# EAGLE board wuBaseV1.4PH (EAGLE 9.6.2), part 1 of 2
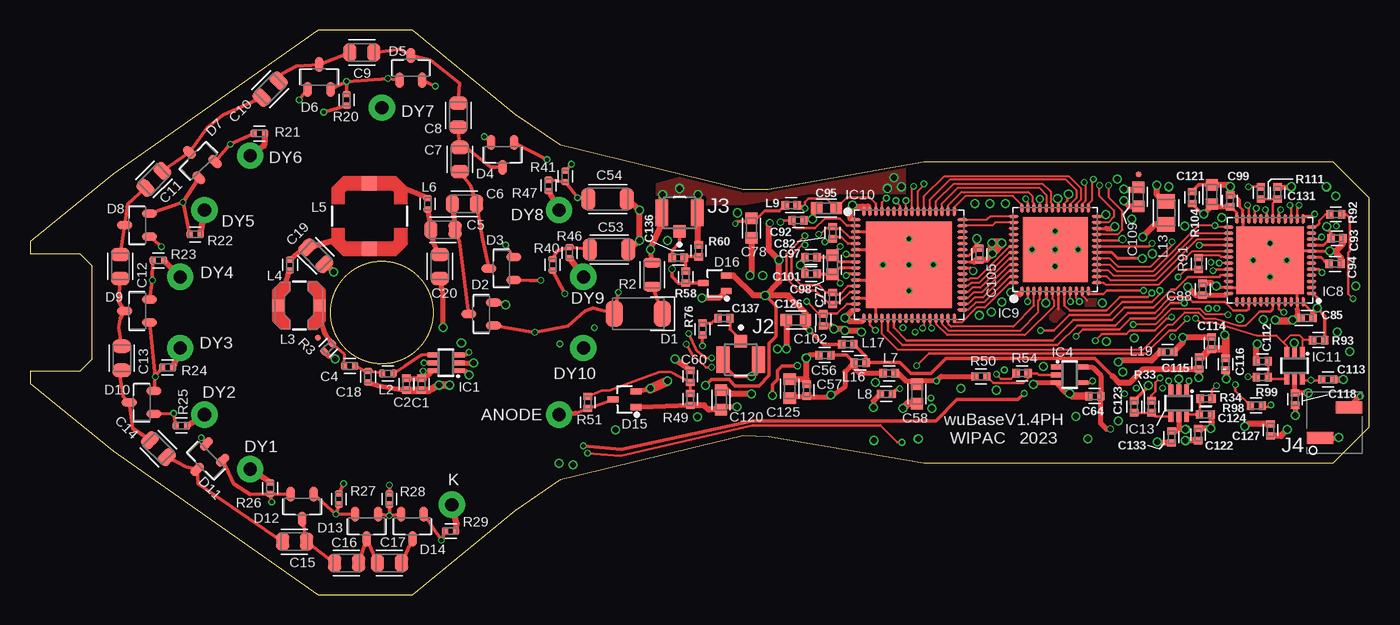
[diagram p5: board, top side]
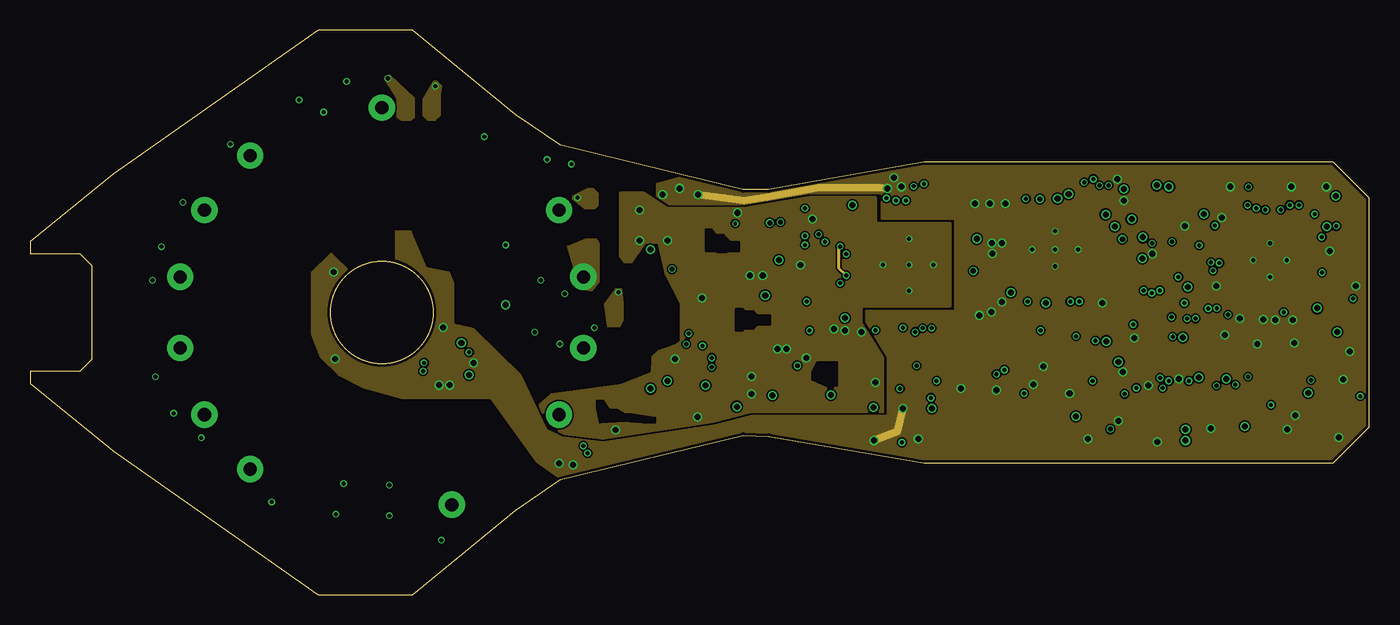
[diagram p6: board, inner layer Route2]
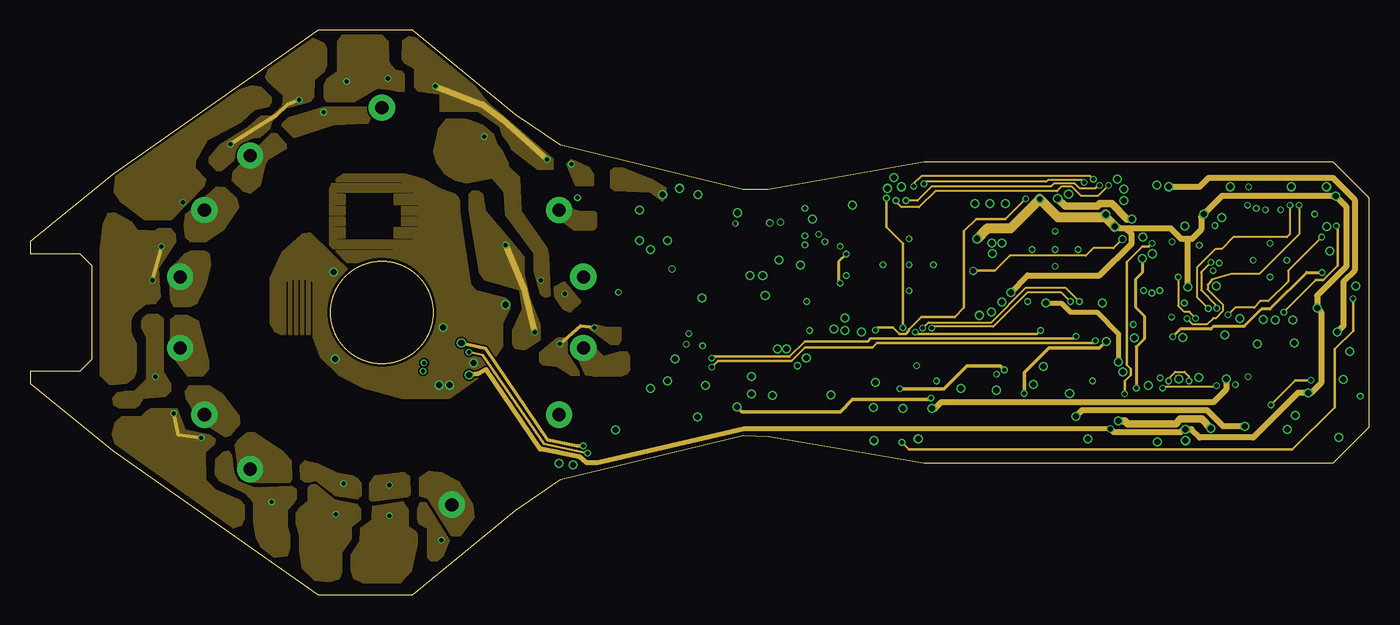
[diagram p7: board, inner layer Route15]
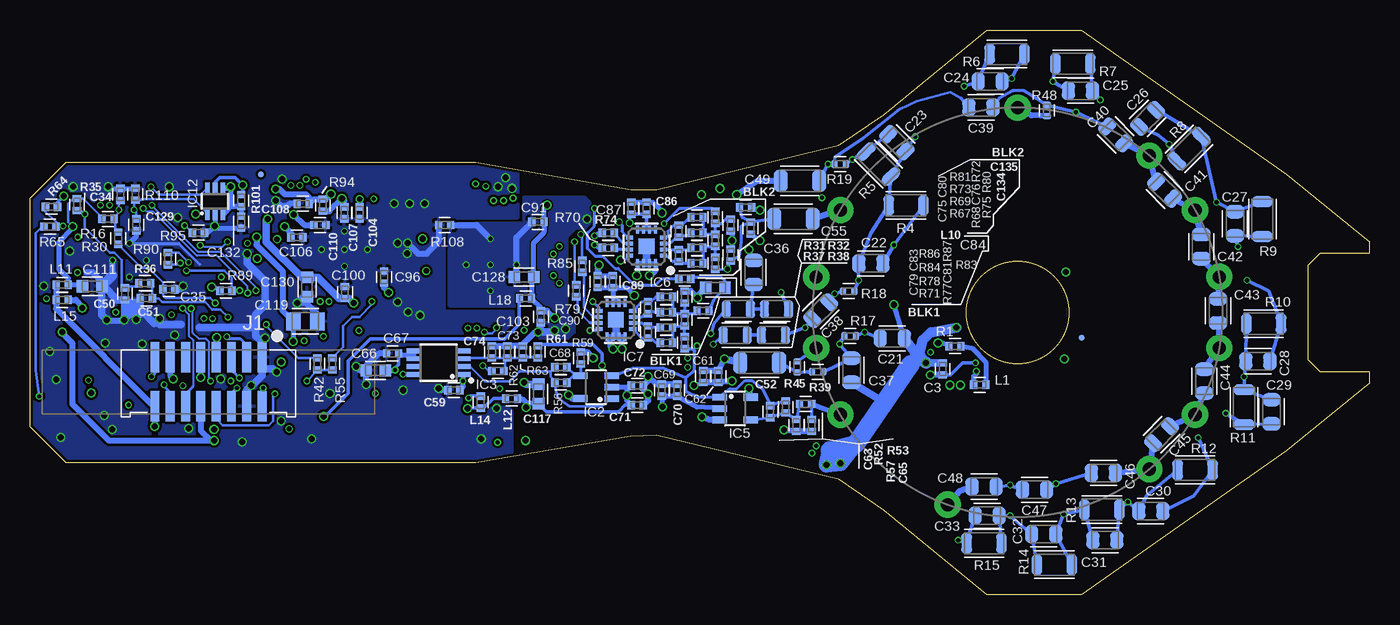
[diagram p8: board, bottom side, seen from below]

Size 111.2 x 46.9 mm. Coordinates in mm from the lower left corner, seen from the top.
Outline: 0,18.55 0,17.55 6.9,11.95 23.9,0 31.75,0 40.31,7.02 44.06,9.57 59.2,13.25 61.33,13.16 74.2,10.95 108.2,10.95 111.2,13.95 111.2,32.95 108.2,35.95 74.2,35.95 61.33,33.65 59.2,33.65 44.06,37.33 40.31,39.88 31.75,46.9 23.9,46.9 6.9,34.95 0,29.35 0,28.35 4.1,28.35 5.1,27.35 5.1,19.55 4.1,18.55 0,18.55
Outline: circle at 29.2,23.45 radius 4.25
Copper layers (1*2*15*16): Top 0.035mm / dielectric 0.23mm / Route2 0.035mm / dielectric 0.93mm / Route15 0.035mm / dielectric 0.23mm / Bottom 0.035mm
Design rules "MF_Standard_4_Layer": minimum track width 5mil, minimum drill 10mil, track to track 5mil, track to pad 5mil, pad to pad 5mil, via to via 5mil, smd to smd 0mil, copper to edge 10mil, drill to drill 10mil, minimum pad ring 4mil, minimum via ring 4mil, stop-mask expansion 2mil, vias tented up to drill 25mil, thermal gap 10mil

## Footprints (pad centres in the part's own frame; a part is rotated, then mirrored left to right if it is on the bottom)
0430-BARE = drill 1.092 pad 2.184: P$1 0,0
C0402 = smd 0.6 x 0.7: 1 -0.5,0; 2 0.5,0
C0402-HV = smd 0.56 x 0.7: 1 -0.47,0; 2 0.47,0
C0805-HV = smd 1.1 x 1.5: 1 -1,0; 2 1,0
C1206-HV = smd 1.165 x 1.815: 1 -1.6,0; 2 1.6,0
C0603 = smd 0.95 x 1: 1 -0.8,0; 2 0.8,0
C0805 = smd 1.2 x 1.5: 1 -1,0; 2 1,0
DO214AC-HV = smd 1.4 x 2.2: A 2,0; C -2,0
SOT23-ROUNDED = smd 1.242 x 0.694: 1 -1.029,0.95; 2 -1.029,-0.95; 3 1.029,0
SC70-3L = smd 0.5 x 0.9: 1 -0.65,-0.95; 2 0.65,-0.95; 3 0,0.95
FIDUCIAL_0.5MM = smd 0.5 x 0.5 bottom: FID_BOT 0,0 | smd 0.5 x 0.5: FID_TOP 0,0
SC70-6L-TI = smd 0.4 x 0.9: 1 -0.65,-1.1; 2 0,-1.1; 3 0.65,-1.1; 4 0.65,1.1; 5 0,1.1; 6 -0.65,1.1
SOT23-5 = smd 0.55 x 1.2: 1 -0.95,-1.3; 2 0,-1.3; 3 0.95,-1.3; 4 0.95,1.3 | smd 0.6 x 1.2: 5 -0.95,1.3
MSOP8 = smd 0.4 x 1.2: 1 -0.975,-2.05; 2 -0.325,-2.05; 3 0.325,-2.05; 4 0.975,-2.05; 5 0.975,2.05; 6 0.325,2.05; 7 -0.325,2.05; 8 -0.975,2.05
SC70-5L-TI = smd 0.4 x 0.9: 1 -0.65,-1.1; 2 0,-1.1; 3 0.65,-1.1; 4 0.65,1.1; 5 -0.65,1.1
LFCSP16 = smd 0.3 x 0.65: 1 -0.75,-1.4; 2 -0.25,-1.4; 3 0.25,-1.4; 4 0.75,-1.4; 9 0.75,1.4; 10 0.25,1.4; 11 -0.25,1.4; 12 -0.75,1.4 | smd 0.65 x 0.3: 5 1.4,-0.75; 6 1.4,-0.25; 7 1.4,0.25; 8 1.4,0.75; 13 -1.4,0.75; 14 -1.4,0.25; 15 -1.4,-0.25; 16 -1.4,-0.75 | smd 1.3 x 1.3: EXP 0,0
UFQFPN48-STMICRO = smd 0.86 x 0.27: 1 -3.435,2.75; 2 -3.435,2.25; 3 -3.435,1.75; 4 -3.435,1.25; 5 -3.435,0.75; 6 -3.435,0.25; 7 -3.435,-0.25; 8 -3.435,-0.75; 9 -3.435,-1.25; 10 -3.435,-1.75; 11 -3.435,-2.25; 12 -3.435,-2.75; 25 3.435,-2.75; 26 3.435,-2.25; 27 3.435,-1.75; 28 3.435,-1.25; 29 3.435,-0.75; 30 3.435,-0.25; 31 3.435,0.25; 32 3.435,0.75; 33 3.435,1.25; 34 3.435,1.75; 35 3.435,2.25; 36 3.435,2.75 | smd 0.27 x 0.86: 13 -2.75,-3.435; 14 -2.25,-3.435; 15 -1.75,-3.435; 16 -1.25,-3.435; 17 -0.75,-3.435; 18 -0.25,-3.435; 19 0.25,-3.435; 20 0.75,-3.435; 21 1.25,-3.435; 22 1.75,-3.435; 23 2.25,-3.435; 24 2.75,-3.435; 37 2.75,3.435; 38 2.25,3.435; 39 1.75,3.435; 40 1.25,3.435; 41 0.75,3.435; 42 0.25,3.435; 43 -0.25,3.435; 44 -0.75,3.435; 45 -1.25,3.435; 46 -1.75,3.435; 47 -2.25,3.435; 48 -2.75,3.435 | smd 5.6 x 5.6: 49 0,0
QFN48-ICE40ULTRA = smd 0.811 x 0.25: 1 -3.451,2.75; 2 -3.451,2.25; 3 -3.451,1.75; 4 -3.451,1.25; 5 -3.451,0.75; 6 -3.451,0.25; 7 -3.451,-0.25; 8 -3.451,-0.75; 9 -3.451,-1.25; 10 -3.451,-1.75; 11 -3.451,-2.25; 12 -3.451,-2.75; 25 3.451,-2.75; 26 3.451,-2.25; 27 3.451,-1.75; 28 3.451,-1.25; 29 3.451,-0.75; 30 3.451,-0.25; 31 3.451,0.25; 32 3.451,0.75; 33 3.451,1.25; 34 3.451,1.75; 35 3.451,2.25; 36 3.451,2.75 | smd 0.25 x 0.811: 13 -2.75,-3.451; 14 -2.25,-3.451; 15 -1.75,-3.451; 16 -1.25,-3.451; 17 -0.75,-3.451; 18 -0.25,-3.451; 19 0.25,-3.451; 20 0.75,-3.451; 21 1.25,-3.451; 22 1.75,-3.451; 23 2.25,-3.451; 24 2.75,-3.451; 37 2.75,3.451; 38 2.25,3.451; 39 1.75,3.451; 40 1.25,3.451; 41 0.75,3.451; 42 0.25,3.451; 43 -0.25,3.451; 44 -0.75,3.451; 45 -1.25,3.451; 46 -1.75,3.451; 47 -2.25,3.451; 48 -2.75,3.451 | smd 5.4 x 5.4: PAD 0,0
QFN64-LTC214X = smd 0.86 x 0.27: 1 -4.435,3.75; 2 -4.435,3.25; 3 -4.435,2.75; 4 -4.435,2.25; 5 -4.435,1.75; 6 -4.435,1.25; 7 -4.435,0.75; 8 -4.435,0.25; 9 -4.435,-0.25; 10 -4.435,-0.75; 11 -4.435,-1.25; 12 -4.435,-1.75; 13 -4.435,-2.25; 14 -4.435,-2.75; 15 -4.435,-3.25; 16 -4.435,-3.75; 33 4.435,-3.75; 34 4.435,-3.25; 35 4.435,-2.75; 36 4.435,-2.25; 37 4.435,-1.75; 38 4.435,-1.25; 39 4.435,-0.75; 40 4.435,-0.25; 41 4.435,0.25; 42 4.435,0.75; 43 4.435,1.25; 44 4.435,1.75; 45 4.435,2.25; 46 4.435,2.75; 47 4.435,3.25; 48 4.435,3.75 | smd 0.27 x 0.86: 17 -3.75,-4.435; 18 -3.25,-4.435; 19 -2.75,-4.435; 20 -2.25,-4.435; 21 -1.75,-4.435; 22 -1.25,-4.435; 23 -0.75,-4.435; 24 -0.25,-4.435; 25 0.25,-4.435; 26 0.75,-4.435; 27 1.25,-4.435; 28 1.75,-4.435; 29 2.25,-4.435; 30 2.75,-4.435; 31 3.25,-4.435; 32 3.75,-4.435; 49 3.75,4.435; 50 3.25,4.435; 51 2.75,4.435; 52 2.25,4.435; 53 1.75,4.435; 54 1.25,4.435; 55 0.75,4.435; 56 0.25,4.435; 57 -0.25,4.435; 58 -0.75,4.435; 59 -1.25,4.435; 60 -1.75,4.435; 61 -2.25,4.435; 62 -2.75,4.435; 63 -3.25,4.435; 64 -3.75,4.435 | smd 7.15 x 7.15: PAD 0,0
3M-45216-220230 = smd 0.737 x 2.54: 1 -4.445,-2.032; 2 -4.445,2.032; 3 -3.175,-2.032; 4 -3.175,2.032; 5 -1.905,-2.032; 6 -1.905,2.032; 7 -0.635,-2.032; 8 -0.635,2.032; 9 0.635,-2.032; 10 0.635,2.032; 11 1.905,-2.032; 12 1.905,2.032; 13 3.175,-2.032; 14 3.175,2.032; 15 4.445,-2.032; 16 4.445,2.032
HIROSE_U.FL-R-SMT-1 = smd 1 x 1.05: 1 0,-1.525 | smd 1.05 x 2.2: 2 1.475,0; 3 -1.475,0
HEADER-SMD-2X1-MINIMUM = smd 1 x 2.2: 1 -1.27,1.2; 2 1.27,-1.2
L0402 = smd 0.6 x 0.7: 1 -0.5,0; 2 0.5,0
L0402-HV = smd 0.56 x 0.7: 1 -0.47,0; 2 0.47,0
LPS4040-REDUCED = smd 1 x 1: 1 -1.7,0; 2 1.7,0
LPS6235-REDUCED = smd 1.2 x 1.2: 1 -2.7,0; 2 2.7,0
L0805 = smd 1.2 x 1.5: 1 -0.953,0; 2 0.953,0
R0402 = smd 0.6 x 0.7: 1 -0.5,0; 2 0.5,0
R0805-HV = smd 0.8 x 1.5: 1 -1,0; 2 1,0
R0402-HV = smd 0.56 x 0.7: 1 -0.47,0; 2 0.47,0
R1206-HV = smd 0.9 x 1.7: 1 -1.45,0; 2 1.45,0

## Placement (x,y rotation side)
ANODE  PAD-0430-BARE  [0430-BARE]  43.92,14.95 0 bottom
C1  1000pF  [C0402]  32.5,17.48 90 top
C2  0.1uF  [C0402]  31.23,17.48 90 top
C3  0.1uF  [C0402]  35.42,18.75 270 bottom
C4  0.1uF  [C0402-HV]  26.53,19 0 top
C5  2200pF/250V  [C0805-HV]  34.28,30.31 0 top
C6  2200pF/250V  [C0805-HV]  36.06,32.47 0 top
C7  2200pF/250V  [C0805-HV]  35.68,36.15 90 top
C8  2200pF/250V  [C0805-HV]  35.55,39.83 90 top
C9  2200pF/250V  [C0805-HV]  27.55,45.04 180 top
C10  2200pF/250V  [C0805-HV]  19.93,41.99 225 top
C11  2200pF/250V  [C0805-HV]  10.28,34.5 225 top
C12  2200pF/250V  [C0805-HV]  7.48,27.26 270 top
C13  2200pF/250V  [C0805-HV]  7.61,19.64 270 top
C14  2200pF/250V  [C0805-HV]  10.66,12.15 315 top
C15  2200pF/250V  [C0805-HV]  21.96,4.4 0 top
C16  2200pF/250V  [C0805-HV]  26.28,2.62 0 top
C17  2200pF/250V  [C0805-HV]  29.84,2.62 0 top
C18  100pF  [C0402-HV]  28.06,18.12 270 top
C19  3900pF/50V  [C0805-HV]  23.74,28.15 315 top
C20  220pF/100V/5%  [C0805-HV]  34.03,27.26 270 top
C21  2200pF/250V  [C0805-HV]  39.61,21.29 180 bottom
C22  2200pF/250V  [C0805-HV]  41.39,27.51 180 bottom
C23  2200pF/250V  [C0805-HV]  39.23,37.55 135 bottom
C24  2200pF/250V  [C0805-HV]  31.49,42.63 0 bottom
C25  2200pF/250V  [C0805-HV]  23.99,41.86 0 bottom
C26  2200pF/250V  [C0805-HV]  18.41,39.58 45 bottom
C27  2200pF/250V  [C0805-HV]  11.17,30.82 270 bottom
C28  2200pF/250V  [C0805-HV]  9.26,19.39 180 bottom
C29  2200pF/250V  [C0805-HV]  8.12,15.19 270 bottom
C30  2200pF/250V  [C0805-HV]  18.15,6.94 180 bottom
C31  2200pF/250V  [C0805-HV]  21.96,4.53 180 bottom
C32  2200pF/250V  [C0805-HV]  27.04,5.04 180 bottom
C33  2200pF/250V  [C0805-HV]  31.74,6.56 180 bottom
C34  0.1uF  [C0402]  103.71,33.24 90 bottom
C35  0.01uF  [C0402]  99.67,25.37 0 bottom
C36  2200pF/250V  [C0805-HV]  51.13,26.77 90 bottom
C37  2200pF/250V  [C0805-HV]  43,18.64 90 bottom
C38  2200pF/250V  [C0805-HV]  45.54,23.59 45 bottom
C39  2200pF/250V  [C0805-HV]  32.25,40.47 0 bottom
C40  2200pF/250V  [C0805-HV]  21.07,38.18 315 bottom
C41  2200pF/250V  [C0805-HV]  17.01,33.61 315 bottom
C42  2200pF/250V  [C0805-HV]  13.96,28.91 270 bottom
C43  2200pF/250V  [C0805-HV]  12.56,23.58 270 bottom
C44  2200pF/250V  [C0805-HV]  13.71,17.73 270 bottom
C45  2200pF/250V  [C0805-HV]  17.26,13.29 225 bottom
C46  2200pF/250V  [C0805-HV]  22.09,10.11 180 bottom
C47  2200pF/250V  [C0805-HV]  27.8,8.72 180 bottom
C48  2200pF/250V  [C0805-HV]  31.99,8.97 180 bottom
C49  10000pF/500V  [C1206-HV]  47.29,34.37 180 bottom
C50  0.1uF  [C0402]  103.33,24.99 270 bottom
C51  0.01uF  [C0402]  101.55,24.61 180 bottom
C52  10000pF/500V  [C1206-HV]  50.62,19.27 0 bottom
C53  10000pF/500V  [C1206-HV]  48.08,28.67 0 top
C54  10000pF/500V  [C1206-HV]  47.96,32.86 0 top
C55  10000pF/500V  [C1206-HV]  47.83,31.21 180 bottom
C56  0.1uF  [C0402]  65.99,19.91 180 top
C57  1000pF  [C0402]  64.47,16.99 90 top
C58  1uF  [C0603]  73.63,16.68 270 top
C59  0.01uF  [C0402]  76.02,16.99 180 bottom
C60  0.1uF  [C0402]  54.81,18.13 90 top
C61  0.1uF  [C0402]  55.32,18.13 90 bottom
C62  1000pF  [C0402]  54.05,18.13 90 bottom
C63  8pF  [C0402]  49.73,15.21 90 bottom
C64  0.1uF  [C0402]  88.4,16.5 0 top
C65  20pF  [C0402]  46.3,14.07 270 bottom
C66  1uF  [C0603]  82.5,18.64 180 bottom
C67  0.01uF  [C0402]  81.1,20.04 180 bottom
C68  DNL  [C0402]  67.13,18.89 180 bottom
C69  0.1uF  [C0402]  58.75,16.99 90 bottom
C70  1000pF  [C0402]  57.48,16.99 90 bottom
C71  0.1uF  [C0402]  60.78,15.74 0 bottom
C72  1000pF  [C0402]  60.78,17.37 0 bottom
C73  0.1uF  [C0402]  71.58,20.16 90 bottom
C74  1000pF  [C0402]  72.85,20.16 90 bottom
C75  3pF  [C0402]  57.35,28.16 90 bottom
C76  7.5pF  [C0402]  54.31,29.43 90 bottom
C77  7.5pF  [C0402]  66.62,24.61 270 top
C78  1uF  [C0603]  59.89,30.45 270 top
C79  4pF  [C0402]  59.89,21.81 90 bottom
C80  3pF  [C0402]  57.35,30.2 90 bottom
C81  8pF  [C0402]  56.85,22.83 90 bottom
C82  11pF  [C0402]  66.62,30.07 90 top
C83  4pF  [C0402]  59.89,23.85 90 bottom
C84  1uF  [C0603]  54.31,25.5 180 bottom
C85  0.1uF  [C0402]  106.02,22.98 180 top
C86  1000pF  [C0402]  60.02,32.1 90 bottom
C87  0.1uF  [C0402]  61.29,32.1 90 bottom
C88  0.1uF  [C0402]  97.36,25.37 90 top
C89  1000pF  [C0402]  62.81,26.01 90 bottom
C90  0.1uF  [C0402]  64.08,26.01 90 bottom
C91  0.1uF  [C0402]  69.04,30.96 180 bottom
C92  0.1uF  [C0402]  63.76,31.11 0 top
C93  0.1uF  [C0402]  108.51,29.61 0 top
C94  0.1uF  [C0402]  108.36,27.48 0 top
C95  2.2uF  [C0603]  66.12,32.1 180 top
C96  0.1uF  [C0402]  81.81,26.39 90 bottom
C97  0.1uF  [C0402]  64.85,28.04 180 top
C98  2.2uF  [C0603]  66.62,27.4 270 top
C99  0.1uF  [C0402]  99.62,32.71 90 top
C100  0.1uF  [C0402]  85.05,25.11 90 bottom
C101  0.1uF  [C0402]  64.85,26.64 180 top
C102  0.1uF  [C0402]  65.86,22.83 270 top
C103  0.1uF  [C0402]  68.78,23.09 270 bottom
C104  0.1uF  [C0402]  83.84,31.72 270 bottom
C105  0.1uF  [C0402]  78.82,28.29 270 top
C106  0.1uF  [C0402]  89.05,29.69 0 bottom
C107  0.1uF  [C0402]  85.11,31.72 270 bottom
C108  0.1uF  [C0402]  88.54,32.48 180 bottom
C109  1uF  [C0603]  92,33.05 270 top
C110  0.1uF  [C0402]  87.14,30.7 0 bottom
C111  4.7uF  [C0603]  106.04,25.62 180 bottom
C112  100pF  [C0402]  102.31,19.4 180 top
C113  100pF  [C0402]  107.75,17.88 0 top
C114  0.1uF  [C0402]  98.1,20.9 270 top
C115  0.1uF  [C0402]  97.05,19.25 90 top
C116  0.1uF  [C0402]  99.26,19.15 90 top
C117  2.2uF  [C0603]  68.99,16.68 270 bottom
C118  0.1uF  [C0402]  105.03,16.25 270 top
C119  10uF/6.3V  [C0805]  88.34,22.7 0 bottom
C120  2.2uF  [C0603]  57.38,16.17 270 top
C121  4.7uF  [C0603]  98.12,33.24 270 top
C122  0.1uF  [C0402]  96.98,13.31 90 top
C123  100pF  [C0402]  91.67,15.62 90 top
C124  100pF  [C0402]  97.59,14.98 0 top
C125  2.2uF  [C0603]  63.07,17.12 270 top
C126  2.2uF  [C0603]  63.58,22.83 0 top
C127  0.1uF  [C0402]  103,13.69 270 top
C128  4.7uF  [C0603]  70.18,26.39 0 bottom
C129  0.1uF  [C0402]  102.39,30.73 90 bottom
C130  4.7uF  [C0603]  88.22,25.55 270 bottom
C131  0.1uF  [C0402]  103.58,33.37 270 top
C132  0.1uF  [C0402]  93.68,30.96 90 bottom
C133  0.1uF  [C0402]  94.77,13.1 270 top
C134  33pF  [C0402]  51.38,30.45 270 bottom
C135  3pF  [C0402]  51.79,32.17 0 bottom
C136  0.1uF  [C0402]  53.82,27.98 180 top
C137  0.1uF  [C0402]  57.61,22.96 180 top
D1  SMAJ150A  [DO214AC-HV]  50.5,23.34 180 top
D2  BAS101S,215  [SOT23-ROUNDED]  37.45,23.32 180 top
D3  BAS101S,215  [SOT23-ROUNDED]  39.12,27.11 180 top
D4  BAS101S,215  [SOT23-ROUNDED]  39.23,36.53 270 top
D5  BAS101S,215  [SOT23-ROUNDED]  31.61,43.77 90 top
D6  BAS101S,215  [SOT23-ROUNDED]  23.99,43.01 90 top
D7  BAS101S,215  [SOT23-ROUNDED]  13.96,36.02 135 top
D8  BAS101S,215  [SOT23-ROUNDED]  8.88,30.69 180 top
D9  BAS101S,215  [SOT23-ROUNDED]  8.88,23.58 180 top
D10  BAS101S,215  [SOT23-ROUNDED]  9.26,15.96 180 top
D11  BAS101S,215  [SOT23-ROUNDED]  14.59,11.13 225 top
D12  BAS101S,215  [SOT23-ROUNDED]  22.6,7.32 270 top
D13  BAS101S,215  [SOT23-ROUNDED]  27.93,5.67 270 top
D14  BAS101S,215  [SOT23-ROUNDED]  31.74,5.67 270 top
D15  BAV99W,115  [SC70-3L]  49.35,16.23 90 top
D16  BAV99W,115  [SC70-3L]  56.85,25.88 90 top
DY1  PAD-0430-BARE  [0430-BARE]  18.27,10.43 0 bottom
DY2  PAD-0430-BARE  [0430-BARE]  14.48,14.95 0 bottom
DY3  PAD-0430-BARE  [0430-BARE]  12.46,20.5 0 bottom
DY4  PAD-0430-BARE  [0430-BARE]  12.46,26.4 0 bottom
DY5  PAD-0430-BARE  [0430-BARE]  14.48,31.95 0 bottom
DY6  PAD-0430-BARE  [0430-BARE]  18.27,36.47 0 bottom
DY7  PAD-0430-BARE  [0430-BARE]  29.2,40.45 0 bottom
DY8  PAD-0430-BARE  [0430-BARE]  43.92,31.95 0 bottom
DY9  PAD-0430-BARE  [0430-BARE]  45.94,26.4 0 bottom
DY10  PAD-0430-BARE  [0430-BARE]  45.94,20.5 0 bottom
FID1  [FIDUCIAL_0.5MM]  23.89,21.34 0 top
FID2  [FIDUCIAL_0.5MM]  92.03,34.9 0 top
IC1  74LVC1T45DCK  [SC70-6L-TI]  34.53,19.26 90 top
IC2  AD8014ART  [SOT23-5]  64.21,17.24 90 bottom
IC3  MAX9013EUA  [MSOP8]  77.29,19.27 90 bottom
IC4  SN74AUC1G17DCK  [SC70-5L-TI]  86.31,18.26 270 top
IC5  AD8014ART  [SOT23-5]  52.66,15.46 270 bottom
IC6  THS4551IRGT  [LFCSP16]  60.02,28.93 90 bottom
IC7  THS4551IRGT  [LFCSP16]  62.56,22.83 90 bottom
IC8  STM32L552CCU  [UFQFPN48-STMICRO]  102.95,27.78 180 top
IC9  ICE40UP5K-SG48I  [QFN48-ICE40ULTRA]  85.11,28.67 90 top
IC10  LTC2142IUP-12  [QFN64-LTC214X]  72.97,27.4 0 top
IC11  74AUP2G3404GW  [SC70-6L-TI]  104.98,19.02 180 top
IC12  INA199C2DCK  [SC70-6L-TI]  95.84,32.69 0 bottom
IC13  74AUP2G3404GW  [SC70-6L-TI]  95.38,15.91 180 top
J1  HDR-16  [3M-45216-220230]  96.39,17.68 180 bottom
J2  COAX-2GNDU.FL  [HIROSE_U.FL-R-SMT-1]  59,19.53 180 top
J3  COAX-2GNDU.FL  [HIROSE_U.FL-R-SMT-1]  53.92,31.72 0 top
J4  HDR-2-SMD  [HEADER-SMD-2X1-MINIMUM]  108.31,14.3 90 top
K  PAD-0430-BARE  [0430-BARE]  35.01,7.47 0 bottom
L1  MMZ1005S601HTD25  [L0402]  32.35,17.43 0 bottom
L2  MMZ1005A222ETD25  [L0402-HV]  29.71,18.37 180 top
L3  1000uH/LPS4040  [LPS4040-REDUCED]  22.34,24.02 0 top
L4  MMZ1005A222ETD25  [L0402-HV]  21.58,27.39 90 top
L5  10000uH/LPS6235  [LPS6235-REDUCED]  28.18,31.45 270 top
L6  MMZ1005A222ETD25  [L0402-HV]  33.01,32.47 90 top
L7  MMZ1005S601HTD25  [L0402]  71.32,18.39 180 top
L8  MMZ1005S601HTD25  [L0402]  71.09,16.68 180 top
L9  MMZ1005A222ETD25  [L0402]  63.2,32.36 180 top
L10  MMZ1005A222ETD25  [L0402]  56.85,26.26 0 bottom
L11  MMZ1005S601HTD25  [L0402]  108.53,25.75 0 bottom
L12  MMZ1005A222ETD25  [L0402]  71.22,16.3 0 bottom
L13  MLZ2012N101LT  [L0805]  94.31,31.72 270 top
L14  MMZ1005A222ETD25  [L0402]  73.79,16 90 bottom
L15  MMZ1005S601HTD25  [L0402]  108.53,24.48 0 bottom
L16  MMZ1005A222ETD25  [L0402]  68.91,19.27 180 top
L17  MMZ1005A222ETD25  [L0402]  67.89,20.8 180 top
L18  MMZ1005S601HTD25  [L0402]  70.05,24.61 0 bottom
L19  MMZ1005S601HTD25  [L0402]  94.44,20.16 180 top
R1  1  [R0402]  34.41,20.66 0 bottom
R2  1M/150V  [R0805-HV]  51.66,26.59 270 top
R3  390K  [R0402-HV]  24.75,20.53 45 top
R4  200M/200V  [R1206-HV]  38.47,32.34 180 bottom
R5  200M/200V  [R1206-HV]  40.76,35.77 135 bottom
R6  200M/200V  [R1206-HV]  30.09,44.91 0 bottom
R7  200M/200V  [R1206-HV]  24.63,44.1 0 bottom
R8  200M/200V  [R1206-HV]  14.98,37.04 45 bottom
R9  200M/200V  [R1206-HV]  8.88,31.2 270 bottom
R10  200M/200V  [R1206-HV]  8.78,22.51 180 bottom
R11  200M/200V  [R1206-HV]  10.4,15.58 270 bottom
R12  200M/200V  [R1206-HV]  14.47,10.37 180 bottom
R13  200M/200V  [R1206-HV]  22.21,7.07 180 bottom
R14  200M/200V  [R1206-HV]  26.15,2.5 180 bottom
R15  200M/200V  [R1206-HV]  31.99,4.27 180 bottom
R16  1.1M  [R0402]  104.73,31.21 0 bottom
R17  390K  [R0402-HV]  43.1,21.48 180 bottom
R18  390K  [R0402-HV]  43.23,25.21 180 bottom
R19  390K  [R0402-HV]  43.93,35.77 180 bottom
R20  390K  [R0402-HV]  26.28,41.1 270 top
R21  390K  [R0402-HV]  19.04,38.31 0 top
R22  390K  [R0402-HV]  13.71,29.93 0 top
R23  390K  [R0402-HV]  10.66,27.77 0 top
R24  390K  [R0402-HV]  11.42,18.88 0 top
R25  390K  [R0402-HV]  12.56,14.05 0 top
R26  390K  [R0402-HV]  19.93,8.84 90 top
R27  390K  [R0402-HV]  25.64,7.96 90 top
R28  390K  [R0402-HV]  29.84,7.96 90 top
R29  390K  [R0402-HV]  34.91,5.29 0 top
R30  10M  [R0402]  103.89,29.61 270 bottom
R31  47M/150V  [R0805-HV]  52.4,23.72 0 bottom
R32  47M/150V  [R0805-HV]  49.23,23.72 0 bottom
R33  27  [R0402]  93.11,15.61 270 top
R34  27  [R0402]  97.64,16.28 180 top
R35  1.1M  [R0402]  107.32,32.41 270 bottom
R36  10M  [R0402]  101.68,25.88 0 bottom
R37  47M/150V  [R0805-HV]  52.66,21.56 0 bottom
R38  47M/150V  [R0805-HV]  49.48,21.56 0 bottom
R39  390K  [R0402-HV]  45.8,18.51 180 bottom
R40  390K  [R0402-HV]  43.38,27.4 90 top
R41  390K  [R0402-HV]  44.44,34.75 270 top
R42  1K  [R0402]  87.35,19.17 90 bottom
R45  49.9  [R0402-HV]  47.5,18.92 90 bottom
R46  49.9  [R0402-HV]  44.78,28.42 270 top
R47  100K  [R0402-HV]  43.04,33.99 270 top
R48  49.9  [R0402-HV]  26.79,40.21 270 bottom
R49  1K  [R0402]  54.81,16.23 90 top
R50  510  [R0402]  78.94,18.13 180 top
R51  47K  [R0402]  46.3,15.97 270 top
R52  1.2K  [R0402]  48.46,15.59 270 bottom
R53  22  [R0402]  46.81,15.85 0 bottom
R54  270  [R0402]  82.37,18.39 0 top
R55  200  [R0402]  86.11,19.17 90 bottom
R56  1K  [R0402]  67.13,17.62 180 bottom
R57  1K  [R0402]  47.58,14.07 270 bottom
R58  DNL  [R0402]  54.43,26.39 270 top
R59  200  [R0402]  65.48,19.66 90 bottom
R60  56  [R0402]  55.5,28.57 90 top
R61  DNL  [R0402]  69.04,20.16 90 bottom
R62  270K  [R0402]  72.36,18.58 180 bottom
R63  DNL  [R0402]  70.31,20.16 90 bottom
R64  20K  [R0402]  109.42,32.23 180 bottom
R65  1K  [R0402]  109.55,30.58 180 bottom
R67  1.8K  [R0402]  55.83,27.53 180 bottom
R68  750  [R0402]  54.31,27.53 90 bottom
R69  330  [R0402]  55.83,28.8 180 bottom
R70  220  [R0402]  63.2,28.8 180 bottom
R71  1.8K  [R0402]  58.37,20.93 180 bottom
R72  2.7K  [R0402]  54.31,31.34 270 bottom
R73  330  [R0402]  55.83,30.07 180 bottom
R74  220  [R0402]  63.2,30.07 180 bottom
R75  430  [R0402]  53.04,28.22 270 bottom
R76  1K  [R0402]  55.83,22.07 90 top
R77  1.2K  [R0402]  56.85,20.93 90 bottom
R78  240  [R0402]  58.37,22.2 180 bottom
R79  220  [R0402]  65.86,25.24 90 bottom
R80  2.2K  [R0402]  53.04,30.7 90 bottom
R81  1.8K  [R0402]  55.83,31.34 180 bottom
R83  2.4K  [R0402]  55.32,23.59 180 bottom
R84  240  [R0402]  58.37,23.47 180 bottom
R85  220  [R0402]  65.36,27.28 90 bottom
R86  1.8K  [R0402]  58.37,24.74 180 bottom
R87  2.4K  [R0402]  56.85,24.74 270 bottom
R89  2.2K  [R0402]  94.95,25.24 0 bottom
R90  1K  [R0402]  99.75,27.91 270 bottom
R91  100  [R0402]  97.03,27.5 90 top
R92  1K  [R0402]  108.41,31.59 180 top
R93  20K  [R0402]  106.99,21.15 0 top
R94  100  [R0402]  86.89,32.36 90 bottom
R95  10K  [R0402]  97.23,30.07 0 bottom
R98  27  [R0402]  101.8,15.72 0 top
R99  27  [R0402]  102.31,18.06 0 top
R101  1  [R0402]  93.68,32.74 270 bottom
R104  100K  [R0402]  96.47,32.99 270 top
R108  0  [R0402]  76.78,30.7 180 bottom
R110  100K  [R0402]  102.46,33.27 90 bottom
R111  100K  [R0402]  102.19,33.37 90 top

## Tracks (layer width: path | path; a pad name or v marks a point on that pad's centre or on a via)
(CDONE)
  Top 0.203: IC9.7 85.36,23.72
  pour Top: 85.4,23.85 85.88,23.36 85.2,22.69 84.95,22.69 84.73,22.91 84.73,23.18
(FPGA_PIN11)
  Top 0.152: 87.78,24.43 87.36,24.85 IC9.11
  pour Top: 87.65,24.56 88.6,24.56 88.6,23.97 87.65,23.97
+VAMP  (via drill 0.35, 0.4, 0.5)
  Top 0.305: v61.04,24.86 61.93,23.97 61.93,21.43 61.37,20.88 61.37,18.21 60.5,17.34 58.55,17.34 58.03,17.86 56.58,17.86 v56.08,17.37 | v64.72,21.94 65.86,20.8 L17.2
  Top 0.406: D15.2 v51.51,17.12
  Top 0.508: v61.04,24.86 62.94,24.86 64.38,23.43 C126.2 64.38,22.29 v64.72,21.94 | v61.04,24.86 62.18,26.01 v62.18,27.78 61.29,28.67 61.29,30.76 v61.42,30.88 | v61.04,24.86 61.02,24.88 60.03,24.88 58.38,26.53 D16.2
  Top 0.813: v51.51,17.12 v52.91,17.75
  Bottom 0.254: IC7.5 IC7.6 IC7.7 IC7.8 | IC7.12 64.07,22.08 64.21,21.94 v64.72,21.94 | v62.18,27.78 61.81,27.78 IC6.12
  Bottom 0.305: 60.02,30.33 IC6.7 IC6.8 | 60.02,30.33 IC6.6 IC6.5 | v61.42,30.88 61.42,31.48 C87.1 C86.1 | 60.02,31.47 60.02,30.33 | C61.1 v56.08,17.37
  Bottom 0.406: C86.1 60.02,31.47 | C90.1 C89.1 | C89.1 62.81,24.68 62.31,24.3 IC7.6 | C89.1 61.68,25.51 v61.04,24.86
  Bottom 0.508: IC5.5 v51.51,17.12 | v52.91,17.75 C62.1 C61.1
+VAMP2  (via drill 0.5)
  Top 0.305: L16.2 67.78,19.91 C56.1
  Top 0.406: C125.2 63.2,16.44 64.42,16.44 C57.1 64.55,16.41 66.3,16.41 v66.5,16.61 66.88,16.73 67.65,17.25 67.65,18.51 L16.2 68.41,18.89 68.88,18.42 70.82,18.42 L7.2
  Bottom 0.508: IC2.5 66.18,16.29 v66.5,16.61
+VDISC  (via drill 0.35)
  Top 0.406: R50.2 75.64,18.13 v75.26,17.75 73.91,17.75 C58.1 73.38,17.73 72.76,17.73 72.11,18.39 L7.1
  Bottom 0.203: v75.26,17.75 75.24,17.73
  Bottom 0.406: IC3.1 75.24,17.73 75.24,17.27 C59.1
-DISCRIM_BUFOUT  (via drill 0.35)
  Top 0.203: v88.22,17.75 88.07,17.61 IC4.4
  Bottom 0.203: v88.22,17.75 87.35,18.62 R42.1 R55.1
-DISCRIM_OUT  (via drill 0.35)
  Top 0.203: v80.24,18.31 80.62,17.93 81.42,17.93 R54.1
  Bottom 0.254: v80.24,18.31 v80.23,18.3 IC3.8
-DISCRIM_OUT_DIVIDER
  Top 0.203: IC4.2 83.77,18.26 83.64,18.39 R54.2 82.87,18 82.47,17.6 79.98,17.6 R50.1
-DISCRIM_OUT_FPGA  (via drill 0.35)
  Top 0.203: IC9.2 82.86,24.39 v82.82,24.36
  Bottom 0.203: v82.82,24.36 82.82,24.1 83.84,23.09 84.47,23.09 85.22,22.34 85.22,20.56 R55.2
-DISCRIM_OUT_MCU  (via drill 0.35)
  Top 0.152: v91.59,22.45 93.42,22.45 94.72,23.75 97.16,23.75 97.61,23.29 99.44,23.29 v99.47,23.26
  Top 0.203: v107.24,29.71 107.06,29.53 IC8.10
  Route15 0.152: 101.63,23.85 100.05,23.85 v99.47,23.26 | v107.24,29.71 104.45,26.92 104.45,26.03 102.8,24.38 102.16,24.38
  Route15 0.203: 102.16,24.38 101.63,23.85
  Bottom 0.203: R42.2 88.94,19.67 91.59,22.32 v91.59,22.45
-VAMP  (via drill 0.35, 0.5)
  Top 0.406: R49.1 50.66,15.58 D15.1 | v58.67,15.62 57.62,15.62 C120.2
  Top 0.508: C120.2 56.33,15.37 55.97,15.73 R49.1
  Route15 0.305: v58.67,15.62 59.1,15.19 67.27,15.19 68.28,16.21 74.67,16.21 v74.79,16.34
  Bottom 0.305: L14.2 74.63,16.5 v74.79,16.34
  Bottom 0.406: IC5.2 55.83,15.59 C70.1 C69.1 58.75,15.69 v58.67,15.62
-VAMP2  (via drill 0.4, 0.5)
  Top 0.305: v63.7,19.02 62.43,19.02 62.05,18.64 62.05,17.88 61.65,17.47 v61.65,16.56
  Top 0.406: L8.2 70.02,16.1 v70.02,15.55
  Bottom 0.305: v63.7,19.02 63.7,20.03 64.47,20.79 68.91,20.79 R61.2 | C71.1 61.8,15.74 62.35,15.19 68.3,15.19 C117.2
  Bottom 0.406: C71.1 61.65,16.11 v61.65,16.56 61.65,17.01 C72.1 61.41,17.24 IC2.2 | v70.02,15.55 70.02,15.96 | L12.2 70.36,16.3 70.02,15.96 | C117.2 69.94,15.88 70.02,15.96
-VDISC  (via drill 0.35)
  Top 0.305: L8.1 72.03,17.12 v72.21,17.12
  Route15 0.305: v80.9,18.66 80.54,19.02 77.8,19.02 75.88,17.1 72.23,17.1 v72.21,17.12
  Bottom 0.305: v80.9,18.66 80.9,18.84 80.6,19.14 C67.1
  Bottom 0.406: C66.1 80.92,18.64 v80.9,18.66 | IC3.5 79.34,19.91 | 79.34,19.91 IC3.6 | C67.1 80.48,19.91 79.34,19.91
ADC1_IN8  (via drill 0.35)
  Top 0.203: v106.66,31.62 106.5,31.47 105.82,31.47 105.7,31.35 IC8.13
  Bottom 0.203: R35.2 106.94,31.91 v106.66,31.62 106.66,30.48 104.6,28.42 104.22,28.42 103.58,27.78 103.58,25.71 C50.1 103.2,25.62 102.44,25.62 R36.1
ADC1_IN12  (via drill 0.35)
  Top 0.203: IC8.17 103.7,31.84 v103.84,31.98
  Bottom 0.203: C34.1 103.84,32.62 v103.84,31.98 103.84,31.72 104.23,31.33 R16.2 104.23,30.96 104.14,30.88 104.14,30.37 R30.1
ADC1_IN15
  Top 0.203: R111.1 C131.2 103.2,32.49 IC8.18
ADC1_IN16  (via drill 0.35)
  Top 0.203: IC8.19 102.7,31.84 v102.57,31.98
  Bottom 0.203: C129.2 102.39,31.8 v102.57,31.98 102.57,32.67 R110.1 102.02,32.77 101.93,32.86 97.64,32.86 96.48,31.71 IC12.1
ADC_!CS
  Top 0.152: 102.11,23.54 100.94,22.37 100.26,22.37 98.42,22.94 97.5,22.94 96.99,23.45 95.88,23.45 94.86,22.43 94.48,22.43 92.42,20.38 72.02,20.38 70.72,21.68 IC10.20
  Top 0.203: IC8.43 103.2,23.72 103.02,23.54 102.11,23.54
ADC_CLKOUT  (via drill 0.45)
  Top 0.203: v90.7,29.54 90.58,29.42 IC9.20
  Top 0.254: IC10.40 78.05,27.15 v78.31,26.89
  Route15 0.152: 80.12,26.91 81.37,28.16 87.65,28.16 88.28,28.8 89.96,28.8
  Route15 0.203: 80.12,26.91 78.33,26.91 v78.31,26.89 | v90.7,29.54 89.96,28.8
ADC_ENC  (via drill 0.35)
  Top 0.203: IC9.35 82.86,32.57 82.67,32.76 v82.67,32.89 | v70.18,21.97 70.16,21.97 69.72,22.4 IC10.18
  Route15 0.203: v82.67,32.89 81,31.21 78.56,31.21 77.55,30.2 77.55,23.85 76.78,23.09 74.02,23.09 72.98,22.05 72.98,21.94 72.7,21.66 72.19,21.66 71.66,22.2 70.41,22.2 v70.18,21.97
ADC_OUT1_0
  Top 0.152: IC9.38 80.14,30.92 79.88,30.67 77.43,30.67 IC10.47
ADC_OUT1_1
  Top 0.152: IC9.37 79.71,31.42 79.44,31.15 IC10.48
ADC_OUT1_2
  Top 0.152: IC9.36 82.36,32.38 81.62,33.12 77.66,33.12 76.72,32.18 IC10.49
ADC_OUT1_3
  Top 0.152: IC10.50 76.22,32.33 77.34,33.45 82.88,33.45 83.21,33.11 83.21,32.68 83.36,32.53 IC9.34
ADC_OUT1_4
  Top 0.152: IC10.51 75.72,32.49 77.04,33.8 83.79,33.8 84.4,33.19 84.4,32.41 84.35,32.36 84.35,32.14 IC9.32
ADC_OUT1_5
  Top 0.152: IC10.52 75.22,32.68 76.68,34.13 84.07,34.13 84.73,33.47 84.73,32.58 84.86,32.45 IC9.31
ADC_OUT1_6
  Top 0.152: IC10.53 74.72,32.84 76.35,34.46 86,34.46 86.87,33.59 86.87,32.96 86.36,32.45 IC9.28
ADC_OUT1_7
  Top 0.152: IC10.54 74.22,33.1 75.9,34.77 86.25,34.77 87.24,33.78 87.24,32.81 86.86,32.43 IC9.27
ADC_OUT1_8  (via drill 0.35)
  Top 0.152: IC10.55 73.72,33.51 74.22,34.01 v74.22,34.13 | IC9.26 87.36,32.45 87.61,32.71 87.61,34.17 v87.52,34.26
  Route15 0.152: v87.52,34.26 87.34,34.44 84.5,34.44 84.37,34.31 74.4,34.31 v74.22,34.13
ADC_OUT1_9  (via drill 0.35)
  Top 0.152: IC10.56 73.22,33.8 v73.36,33.93 | v88.28,34.52 88.16,34.39 88.16,32.75 87.86,32.45 IC9.25
  Route15 0.152: v88.28,34.52 88.03,34.77 73.99,34.77 73.36,34.13 v73.36,33.93
ADC_OUT1_10  (via drill 0.35)
  Top 0.152: IC10.57 v72.72,32.73 v72.72,32.74 | v88.79,34.01 88.79,33.12 90,31.91 90,31.4 89.52,30.92 IC9.23
  Route15 0.152: v88.79,34.01 88.67,34.01 88.41,33.75 87.14,33.75 86.74,34.16 85.01,34.16 84.75,33.91 74.86,33.91 73.69,32.74 v72.72,32.74
ADC_OUT1_11  (via drill 0.35)
  Top 0.152: IC10.58 72.22,32.31 71.88,32.65 v71.88,32.74 | v89.55,34.01 89.55,32.99 90.7,31.85 90.7,30.32 90.3,29.92 IC9.21
  Route15 0.152: v89.55,34.01 88.67,33.12 87.27,33.12 86.51,33.88 85.62,33.88 85.26,33.52 75.16,33.52 73.81,32.18 72.36,32.18 71.88,32.66 v71.88,32.74
ADC_OUT2_0  (via drill 0.35)
  Top 0.152: IC10.27 74.22,22.25 v74.12,22.14 | v87.12,24.36 86.86,24.61 IC9.10
  Route15 0.152: v74.12,22.14 74.6,22.63 79.83,22.63 82.7,25.5 85.97,25.5 v87.12,24.36
ADC_OUT2_1  (via drill 0.35)
  Top 0.152: IC10.28 74.72,22.48 74.86,22.35 v74.86,22.14 | v86.38,24.36 86.36,24.38 IC9.9
  Route15 0.152: v86.38,24.36 85.62,25.12 82.82,25.12 79.98,22.27 74.98,22.27 v74.86,22.14
ADC_OUT2_2
  Top 0.152: IC10.29 75.22,22.49 76.15,21.56 82.59,21.56 84.98,23.95 84.98,24.46 84.86,24.59 IC9.6
ADC_OUT2_3
  Top 0.152: IC10.30 75.72,22.49 76.3,21.92 82.16,21.92 83.71,23.47 83.71,24.44 83.86,24.59 IC9.4
ADC_OUT2_4
  Top 0.152: IC10.31 76.22,22.53 76.48,22.27 81.63,22.27 83.36,24 IC9.3
ADC_OUT2_5
  Top 0.152: IC10.32 76.72,22.75 76.85,22.62 77.36,22.62 78.58,23.84 79.26,23.84 81.34,25.92 IC9.48
ADC_OUT2_6
  Top 0.152: IC10.33 77.88,23.65 78.52,24.29 79.2,24.29 81.34,26.42 IC9.47
ADC_OUT2_7
  Top 0.152: IC10.34 77.88,24.15 78.42,24.69 79.09,24.69 81.33,26.92 IC9.46
ADC_OUT2_8
  Top 0.152: IC10.35 77.88,24.65 78.34,25.11 79.01,25.11 81.32,27.42 IC9.45
ADC_OUT2_9
  Top 0.152: IC10.36 77.88,25.15 78.23,25.51 78.9,25.51 81.31,27.92 IC9.44
ADC_OUT2_10
  Top 0.152: IC10.37 77.88,25.65 78.14,25.91 78.79,25.91 81.3,28.42 IC9.43
ADC_OUT2_11
  Top 0.152: IC10.38 77.92,26.15 78.05,26.28 78.65,26.28 81.3,28.92 IC9.42
AGND  (via drill 0.35, 0.5)
  Top 0.254: IC10.6 71.72,28.65 | 71.72,28.65 IC10.PAD 71.72,26.15 | IC10.11 71.72,26.15 | IC10.3 70.22,30.15 71.72,28.65 | IC10.19 70.22,24.65 | 70.22,24.65 71.72,26.15 | IC10.14 70.22,24.65
  Top 0.305: J2.2 57.53,19.15 58.55,18.13 v59.89,18.13
  Top 0.406: C97.2 64.35,27.92 63.96,27.53 v63.96,27.4 v63.97,27.4 64.35,27.02 C101.2 | C95.2 65.05,31.89 65.05,31.29 v64.97,31.21 64.36,31.21 C92.2 | C56.2 64.67,19.91 v64.44,19.68
  Top 0.508: J2.3 60.48,18.72 v59.89,18.13 | C125.1 64.44,17.92 | 64.44,17.92 64.47,17.92 64.47,17.59 64.56,17.49 C57.2 | 64.44,17.92 v64.44,19.68 | C78.2 59.89,26.64 v59.77,26.51 | C102.2 66.5,22.33 v66.75,22.08 v66.75,22.07 67.51,22.07 v67.64,21.94 68.91,21.94 v69.04,21.81 | C126.1 62.81,22.76 v62.81,20.42 | C60.2 v53.54,19.58 | D16.1 57.23,24.66 v55.78,24.66 | C120.1 57.89,16.97 58.2,16.66 v59.89,16.66 | C54.2 v50.61,31.96 v50.61,29.42 C53.2
  Bottom 0.305: 62.05,21.43 IC7.16 | IC7.13 63.07,21.43
  Bottom 0.406: v59.77,26.51 59.65,26.51 59.27,26.89 IC6.16 IC6.15 60.02,27.53 IC6.14 IC6.13 60.77,26.77 60.83,26.71 v60.83,26.51 | R75.1 52.91,28.84 v52.91,29.43 52.91,30.08 R80.1 | v58.75,31.72 58.75,31.85 59.5,32.6 C86.2 C87.2 | v62.81,20.42 63.07,20.67 63.07,21.43 IC7.14 62.56,21.43 IC7.15 62.05,21.43 v62.05,20.42 | C90.2 C89.2 | C134.2 v50.61,29.42 | C135.2 v50.61,31.96
  Bottom 0.508: C74.2 C73.2 R63.2 70.31,20.8 69.29,21.81 v69.04,21.81 | v63.96,27.4 64.08,27.28 C90.2 | C91.2 70.82,29.68 v70.82,27.4 70.82,26.55 C128.1 | 68.78,21.81 C103.2 | R108.1 74.12,30.7 v72.97,29.56 | C70.2 C69.2 59.25,17.49 v59.89,18.13 59.89,17.76 C72.2 60.28,17.05 v59.89,16.66 59.89,16.13 C71.2 | IC5.3 54.78,14.54 v55.4,14.75 | C65.2 R57.2 v48.59,13.69 | R59.2 64.92,20.16 v64.44,19.68 | C61.2 C62.2 v53.54,19.58 | R87.1 56.36,25.24 v55.78,24.66 55.78,24.82 C84.2
  Bottom 0.61: IC7.EXP 62.56,21.43 | 60.02,27.53 IC6.EXP | 68.78,21.81 67.77,21.81 v67.64,21.94 | C52.1 v53.54,19.58 | C117.1 70.04,17.48 v70.18,17.62
  other vias: 72.97,27.4 75.01,27.4 72.97,25.24
  pour Route2 (isolate 0.127, rank 2): 48.97,33.34 48.97,28.16 49.35,27.66 49.9,27.64 51.04,29.29 52.19,29.29 52.78,26.64 54.05,24.23 54.05,21.05 53.54,20.67 52.15,20.16 51.68,19.77 51.64,18.39 49.1,17.37 43.26,16.61 42.24,15.72 43,13.94 44.27,13.31 47.45,12.92 56.72,14.32 59.59,15.06 70.83,15.09 70.82,19.7 69.04,22.5 69.04,23.97 76.4,23.97 76.4,30.83 70.22,30.83 70.22,32.98 64.63,32.98 59.95,32.23 59.28,32.1 52.95,32.09 50.92,33.36 49.01,33.36
  cutout Route2: 66.34,17.24 67.01,17.37 67.01,19.27 65.35,19.27 64.97,18.51 64.97,17.88
  cutout Route2: 61.42,23.21 60.4,23.21 60.07,23.54 59.31,23.54 59.13,23.72 58.62,23.72 58.62,21.94 59.13,21.94 59.31,22.12 60.07,22.12 60.4,22.45 61.42,22.45
  cutout Route2: 58.88,29.31 58.17,29.31 57.58,29.89 57,29.89 56.57,30.32 56.13,30.32 56.13,28.55 57,28.55 57.09,28.45 57.83,28.45 57.9,28.53 58.88,28.55
  pour Bottom (isolate 0.127): 76.4,24 68.91,24 68.91,21.31 66.5,21.31 65.99,21.81 65.99,22.7 66.62,23.34 66.62,29.69 65.86,30.45 65.1,30.45 64.72,30.83 64.72,32.61 65.1,32.99 70.23,32.99 70.23,30.83 76.4,30.83
  cutout Route2: 48.72,15.34 49.35,14.96 49.99,14.96 51.89,14.7 51.89,14.32 50.88,14.32 49.35,14.45 47.32,14.32 47.07,15.46 47.07,16.1 47.58,16.1 48.08,15.34
AMP1_INM
  Bottom 0.254: IC5.4 C63.1 R52.2 R57.1 R53.1
AMP2_INM
  Bottom 0.254: IC2.4 65.93,18.19 C68.1 | R56.1 66.06,18.19 IC2.4 | IC2.4 65.48,18.22 R59.1
AMP_VCM1  (via drill 0.4)
  Top 0.203: v62.31,30.96 62.31,31.06 62.34,31.09 63.24,31.09 | IC10.2 67.82,30.65 67.22,31.25 65.99,31.25 65.17,30.43 63.62,30.43 63.24,30.81 63.24,31.09 | C92.1 63.24,31.09
  Bottom 0.254: IC6.9 61.55,29.68 62.06,30.18 62.06,30.71 v62.31,30.96
AMP_VCM2  (via drill 0.35)
  Top 0.203: IC10.15 67.82,24.15 67.01,23.34 65.9,23.34 C102.1 65.51,23.33 v64.48,24.36
  Bottom 0.254: IC7.9 63.96,23.84 v64.48,24.36
ANODE
  Top 0.254: D15.3 R51.2 45.29,15.08
  Top 0.406: ANODE.P$1 45.29,15.08
  Bottom 0.254: R53.2 46.3,15.08 C65.1
  Bottom 0.406: R53.2 ANODE.P$1
ANODE_AMP_OUTN  (via drill 0.35)
  Top 0.203: IC10.5 67.92,29.15 67.35,29.73 66.78,29.73 C82.1 66.51,29.57 66.24,29.31 v65.99,29.31
  Bottom 0.203: v65.99,29.31 65.99,25.84 R79.2
ANODE_AMP_OUTP  (via drill 0.35)
  Top 0.203: v65.48,29.94 65.61,29.94 66.11,30.44 66.5,30.44 C82.2 66.75,30.44 66.75,30.41 67.3,30.41 68.06,29.65 IC10.4
  Bottom 0.203: v65.48,29.94 65.36,29.82 R85.2
ANODE_PREAMP_OUT  (via drill 0.35)
  Top 0.254: v55.83,20.67 R76.1
  Bottom 0.254: 56.03,20.24 56.03,18.61 56.77,18.06 | IC2.3 62.66,18.19 61.13,18.83 58.94,18.83 58.62,18.82 56.77,18.06 | 56.77,18.06 56.77,16.93 55.75,16.43 IC5.1 53.08,17.1 52.57,17.1 51.83,17.79 51.3,17.79 50.41,17.1 C63.2 R52.1 | v55.83,20.67 56.08,20.43 56.22,20.43
  Bottom 0.305: 56.03,20.24 56.22,20.43 R77.1
BIAS_FILT
  Top 0.203: R51.1 47.49,16.97 48.12,16.97 49.77,17.61 52.27,18.51 53.16,18.51 C60.1
  Top 0.254: R49.2 C60.1
BOOT0  (via drill 0.35)
  Top 0.203: IC8.44 103.7,23.73 103.96,23.47 v104.09,23.47
  Route15 0.203: v104.09,23.47 106.76,26.13 107.39,26.13 108.59,27.33 108.59,30.5 v108.46,30.63
  Bottom 0.203: v108.46,30.63 108.51,30.58 R65.1 109.05,30.96 109.92,31.83 R64.2
BOOT_CONTROL  (via drill 0.35)
  Top 0.203: 109.49,15.59 J4.2
  Top 0.406: v110.44,16.48 109.49,15.59
  Bottom 0.203: v110.44,16.48 110.73,18.62 110.73,30.05 110.21,30.58 R65.2
CH1COAX
  Top 0.254: C137.1 58.11,22.07 59,21.17 J2.1
CH1COAX_DC
  Top 0.254: R76.2 56.59,22.57 56.98,22.96 C137.2
CH2COAX
  Top 0.305: C136.2 53.32,28.65 53.92,29.25 J3.1
CH2COAX_DC
  Top 0.305: R58.1 54.43,27.87 C136.1 54.41,28.07 R60.1
CLK20M_N  (via drill 0.35)
  Top 0.254: IC8.5 107,27.03 v107.27,26.77
  Route15 0.254: v94.87,21.43 95.49,22.06 98.04,22.06 98.3,22.31 100.83,22.31 102.24,23.72 102.95,23.72 106,26.77 v107.27,26.77
  Bottom 0.254: J1.3 93.22,20.72 93.78,21.28 94.72,21.28 v94.87,21.43
CLK20M_P  (via drill 0.35, 0.5)
  Top 0.254: IC9.18 89.8,28.42 90.32,27.91 v92.35,27.91
  Route15 0.254: v92.35,27.91 92.35,26.77 91.77,26.19 91.77,23.91 92.51,23.17 92.51,21.26 91.85,20.6 v91.85,17.17
  Bottom 0.406: J1.2 91.9,15.7 91.9,17.12 v91.85,17.17
CW_1_KB
  Top 0.305: D12.3 C15.2 C16.1
CW_2_1
  Top 0.305: C14.2 12.94,10.62 D11.3 13.96,9.23 C15.1
CW_3_2
  Top 0.305: C13.2 7.48,17.99 7.74,16.46 D10.3 8.5,13.8 C14.1
CW_4_3
  Top 0.305: C12.2 7.36,24.34 D9.3 7.48,22.94 7.36,22.18 C13.1
CW_5_4
  Top 0.305: C11.2 8.12,32.47 D8.3 C12.1
CW_6_5
  Top 0.305: C10.2 15.99,39.83 14.72,38.82 D7.3 C11.1
CW_7_6
  Top 0.305: C9.2 D6.3 22.09,43.9 20.95,43.26 C10.1
CW_8_7
  Top 0.305: C9.1 30.72,45.29 D5.3 33.26,44.41 35.68,42.5 C8.2
CW_9_8
  Top 0.305: D4.3 38.22,35.52 36.31,37.04 C7.2 C8.1
CW_10_9
  Top 0.305: D3.3 37.58,29.55 C6.2 36.57,33.99 C7.1
CW_A_10
  Top 0.305: D2.3 35.68,29.29 C5.2
  Top 0.406: C6.1 C5.2
CW_KA_K
  Top 0.305: C17.2 D14.3
CW_KB_KA
  Top 0.305: C16.2 D13.3 C17.1
DISCRIM_IN+
  Bottom 0.203: IC3.2 74.66,18.95 73.44,17.73 71.36,17.73 70.56,18.54 67.98,18.54 | IC2.1 63.74,15.63 66.41,15.63 66.88,15.97 67.39,16.48 67.59,17.05 R56.2 67.63,17.78 67.98,18.13 67.98,18.54 | 67.98,18.54 C68.2
DISCRIM_IN-
  Bottom 0.203: C73.1 C74.1 75.18,19.66 IC3.3 | C73.1 R63.1 | R62.1 71.75,18.7 71.75,19.5 C73.1
  Bottom 0.254: R63.1 70.24,19.73 69.1,19.73 R61.1
DISCRIM_LEVEL  (via drill 0.35)
  Top 0.203: IC8.14 105.2,32.23 105.32,32.36 v105.36,32.36 | v73.61,19.02 74.62,20.03 92.66,20.03 94.59,21.97 95.12,21.97 96.06,22.91 v96.06,22.93
  Route15 0.152: v96.06,22.93 96.55,22.45 97.72,22.45 98.22,22.96 98.43,22.96 99.03,23.55 99.03,24.11 97.78,25.36 97.78,25.74 98.14,26.19 99.72,26.64 102.06,26.64 105.36,29.94 v105.36,32.36
  Bottom 0.203: v73.61,19.02 73.55,19.02 73.12,18.58 R62.2
DRV_FILT
  Top 0.254: L2.2 28.69,18.46 C18.1 27.73,18.59 C4.2
DRV_L1INP
  Top 0.254: C4.1 26.1,19.98 R3.2
  Top 0.406: R3.2 24.5,21.67 24.04,23.15 L3.2
DRV_L1OUT
  Top 0.406: L3.1 20.52,24.15 21.4,26.46 L4.1
DRV_L2INP
  Top 0.406: L4.2 22.25,28.4 22.74,28.66 C19.1
  Top 0.508: C19.1 25.15,29.43 25.99,29 L5.2
DRV_L2OUT
  Top 0.406: L6.2 31.11,33.74 L5.1
DRV_OUT
  Top 0.406: C20.1 33.52,29.16 C5.1 L6.1
DRV_SQUARE
  Top 0.254: IC1.4 32.52,19.91 31.07,18.97 L2.1
DY1
  Top 0.508: R26.2 DY1.P$1
  Bottom 0.508: C46.1 DY1.P$1 C45.2
  pour Route15 (no thermals): 21.71,9.61 21.68,11.11 21.07,11.77 18.66,13.42 18.02,13.42 17.26,12.78 17.03,12.4 17.29,10.62 18.53,9.35 21.58,9.35
DY1A  (via drill 0.35)
  Top 0.305: D11.1 16.88,9.23 18.28,8.34 R26.1 | R26.1 D12.2 | R26.1 v20.06,7.7
  Bottom 0.305: R12.2 18.53,8.21 C30.2 v20.06,7.7 R13.1 C31.1
  pour Route15: 22.09,8.72 21.71,8.97 18.66,8.84 17.26,9.35 16.88,10.11 16.75,11.51 16.5,11.89 15.99,11.77 15.41,11.18 15.38,10.04 15.74,9.48 17.9,8.46 18.56,7.7 18.56,6.05 18.79,4.78 19.17,4.02 20.31,3.13 21.33,3.26 21.55,3.89 21.55,4.98 21.33,5.62 21.33,7.07 21.83,7.57 22.09,7.96
DY2
  Top 0.508: R25.2 DY2.P$1
  Bottom 0.508: C45.1 DY2.P$1 C44.2
  pour Route15 (no thermals): 12.87,16.85 12.94,16.34 13.88,14.81 14.59,14.18 16.25,13.16 16.6,13.29 17.39,14.18 17.36,14.81 15.99,16.59 14.85,17.3 13.2,17.3
DY2A  (via drill 0.35)
  Top 0.305: D11.2 v14.21,13.04 | D10.1 v11.93,15.07 R25.1
  Route15 0.305: v11.93,15.07 12.31,13.29 v14.21,13.04
  Bottom 0.305: v14.21,13.04 R12.1 14.59,8.21 C30.1 | v11.93,15.07 R11.2 C29.2
  pour Route15: 17.39,7.83 17.74,7.45 17.74,6.3 17.52,5.8 16.88,5.54 7.1,12.53 6.85,13.29 7.1,14.31 7.61,14.79 9.26,14.79 9.64,15.19 10.02,15.45 12.18,15.45 12.82,13.67 14.85,13.29 15.36,12.88 15.23,12.5 14.49,11.82 14.52,9.56 15.36,8.72
DY3
  Top 0.508: R24.2 DY3.P$1
  Bottom 0.508: C43.2 DY3.P$1 C44.1
  pour Route15 (no thermals): 13.07,18.19 14.34,18.19 14.82,18.75 14.82,19.39 13.96,22.69 13.07,23.17 12.05,23.17 11.67,22.81 11.67,20.02
DY3A  (via drill 0.35)
  Top 0.305: D9.1 v10.4,18.12 | R24.1 v10.4,18.12 | D10.2 v10.4,18.12
  Bottom 0.305: R10.2 C28.2 v10.4,18.12 R11.1 C29.1
  pour Route15: 10.58,23.25 9.77,23.25 9.39,22.94 9.26,22.69 9.26,22.18 9.67,21.42 9.67,17.86 8.63,16.85 7.86,16.85 7.23,16.72 6.87,16.31 6.95,15.8 7.41,15.58 8.68,15.58 9.06,15.8 9.39,16.34 11.24,16.52 11.67,16.97 11.67,17.48 11.04,18.5 11.06,22.92
DY4
  Top 0.508: R23.2 DY4.P$1
  Bottom 0.508: C42.2 DY4.P$1 C43.1
  pour Route15 (no thermals): 11.67,24.47 11.93,23.98 13.32,23.98 13.83,24.21 14.59,25.74 14.98,27.39 14.85,28.28 14.47,28.5 13.32,28.5 12.82,28.28 11.55,26.88
DY4A  (via drill 0.35)
  Top 0.305: R23.1 v10.15,26.12 D9.2 | v10.91,28.91 D8.1
  Route15 0.305: v10.91,28.91 v10.15,26.12
  Bottom 0.305: C28.1 R10.1 8.37,25.23 v10.15,26.12 | R9.2 C27.2 v10.91,28.91
  pour Route15: 9.52,24.14 10.4,24.21 10.79,24.72 10.63,27.13 12.08,29.32 12.05,29.93 11.67,30.38 10.73,30.41 10.4,30.18 8.91,30.26 8.45,30.89 6.97,31.7 6.47,31.63 6.09,30.74 5.83,28.66 5.83,18.24 6.59,17.48 7.99,17.61 8.63,18.12 8.83,18.62 8.83,20.78 8.37,21.8 8.37,22.81 8.63,23.45
DY5
  Top 0.508: R22.2 DY5.P$1
  Bottom 0.508: C42.1 DY5.P$1 C41.2
  pour Route15 (no thermals): 17.11,32.92 17.26,32.21 15.99,30.31 14.59,29.32 13.32,29.32 12.94,29.67 12.82,30.69 12.94,31.58 15.48,33.86 16.17,33.81
DY5A  (via drill 0.35)
  Top 0.305: R22.1 v12.69,32.59 | D8.2 v12.69,32.59 | D7.1 v12.69,32.59
  Bottom 0.305: R9.1 C27.1 v12.69,32.59 R8.2 C26.2
  pour Route15: 17.54,39.3 18.66,40.34 19.8,40.59 20.03,40.9 20.01,41.31 19.17,42.12 18.41,42.25 17.26,41.86 7.1,34.75 6.97,33.48 7.48,32.72 9.52,31.22 11.78,31.22 14.47,33.99 14.59,34.5 13.71,35.39 13.71,36.02 14.72,37.8
DY6
  Top 0.508: R21.2 19.42,37.29 DY6.P$1
  Bottom 0.508: C41.1 DY6.P$1 C40.2
  pour Route15 (no thermals): 16.88,35.13 20.06,38.31 20.44,38.31 21.2,37.42 21.2,37.04 19.67,36.15 19.42,35.64 19.04,33.99 18.28,33.36 17.72,33.51 16.83,34.4
DY6A  (via drill 0.35)
  Top 0.305: D6.1 v22.34,41.1 | R21.1 v16.63,37.42 D7.2
  Route15 0.305: v16.63,37.42 20.44,39.83 21.33,40.72 v22.34,41.1
  Bottom 0.305: R7.2 C25.2 v22.34,41.1 | C26.1 17.52,38.18 v16.63,37.42 R8.1
  pour Route15: 15.74,37.29 14.85,36.28 14.85,35.9 15.48,35.26 15.86,35.26 16.88,36.15 17.26,37.29 18.28,37.93 19.04,38.05 19.93,38.82 20.06,39.33 21.28,40.47 23.23,40.98 23.56,41.36 23.59,42.8 24.4,43.54 24.63,44.02 24.63,45.29 24.4,45.78 23.48,46.18 19.8,43.64 19.55,43.01 19.8,42.63 21.07,41.48 20.97,40.59 20.06,39.71 19.17,39.71 18.15,38.82
DY7
  Bottom 0.508: R48.2 28.06,39.83 DY7.P$1
DY7A  (via drill 0.35)
  Top 0.305: D5.1 v29.71,42.88 v26.28,42.63 | v26.28,42.63 D6.2 | R20.1 v26.28,42.63
  Bottom 0.305: C24.2 v29.71,42.88 R6.2 | C25.1 v26.28,42.63 R7.1
  pour Route15: 24.4,42.3 24.4,41.36 24.63,40.98 26.91,40.98 28.82,42.12 29.96,41.99 30.47,41.86 31.05,41.86 31.05,43.21 30.83,43.47 30.34,43.52 29.78,44.2 29.73,45.93 29.23,46.44 25.9,46.44 25.52,45.93 25.52,43.39 24.63,42.75
  pour Route2: 29.45,42.88 30.47,41.23 30.47,39.71 30.85,39.45 31.61,39.45 31.87,39.71 31.87,41.23 29.84,43.13
DY7B  (via drill 0.35)
  Top 0.305: v24.37,40.09 R20.2
  Bottom 0.254: R48.1 28.69,41.86 29.58,41.86 30.72,41.23
  Bottom 0.305: C40.1 v24.37,40.09 R48.1 | 30.72,41.23 C39.2
  pour Route15 (no thermals): 21.45,39.58 20.95,39.07 20.95,38.94 21.83,38.05 22.09,38.05 25.26,39.07 28.06,39.2 28.31,39.71 27.93,40.47 24.37,40.47
DY8
  Top 0.508: R47.2 DY8.P$1
  Bottom 0.508: DY8.P$1 C55.1
  pour Route15 (no thermals): 46.98,31.7 46.98,30.56 46.73,30.31 45.2,30.31 43.55,31.45 43.8,32.34 45.71,31.83 46.85,31.83
DY8_AMP_IN  (via drill 0.4)
  Top 0.305: v53.29,27.05 53.29,26.41 53.84,25.86 54.41,25.86 R58.2 55.8,25.89 55.85,25.84
  Top 0.406: 55.85,25.84 D16.3
  Bottom 0.254: C135.1 52.06,31.32 C134.1 52.19,30.56 52.19,29.29 52.34,28.1 R75.2 v53.29,27.05 R68.1
  Bottom 0.305: C55.2 49.71,31.19 C134.1
DY8A  (via drill 0.35)
  Top 0.305: D5.2 v33.64,42.25 | D4.1 v42.92,36.15
  Route15 0.508: v33.64,42.25 37.58,40.72 39.23,39.45 v42.92,36.15
  Bottom 0.305: v33.64,42.25 C24.1 R6.1 | R19.1 v42.92,36.15 R5.2 C23.2
  pour Route15: 34.03,40.21 37.2,40.21 38.98,38.94 39.23,38.18 39.74,37.55 39.97,37.04 42.15,35.39 43.42,35.39 43.42,36.15 38.09,40.72 36.31,43.01 32.38,46.18 31.49,46.31 30.93,45.93 30.9,44.53 31.08,44.2 31.94,43.72 31.94,42.2 32.22,41.86 34.03,41.61
  pour Route2: 33.52,42.63 32.63,41.1 32.63,39.83 33.01,39.45 33.64,39.45 34.03,39.83 34.03,41.48 34.15,42.25 33.77,42.63
DY8B  (via drill 0.35)
  Top 0.305: R41.1 v44.95,35.77
  Bottom 0.203: 38.98,40.34 37.58,40.98 34.79,41.74 33.9,41.23
  Bottom 0.254: 38.98,40.34 42.03,37.93 44.31,36.4 44.4,36.28 R19.2
  Bottom 0.305: R19.2 v44.95,35.77 C49.1 | C39.1 33.9,41.23
  pour Route15: 44.95,36.15 46.34,35.52 46.73,34.88 46.73,33.99 45.33,33.99 44.57,35.77
DY8C  (via drill 0.35)
  Top 0.305: R47.1 R41.2 v45.46,32.98 C54.1
  pour Route2: 45.08,33.1 46.34,33.74 46.73,33.74 47.11,33.36 47.11,32.34 46.85,32.09 46.09,32.09 45.08,32.85
DY9
  Top 0.508: R46.2 DY9.P$1
  pour Route2 (no thermals): 47.19,29.18 47.19,26.01 46.56,25.24 45.67,25.5 44.65,28.93 46.18,29.56 46.94,29.56
DY9_AMP_OUTN  (via drill 0.35)
  Top 0.203: IC10.12 67.92,25.65 67.22,24.95 66.78,24.95 C77.1 66.09,25.11 65.48,25.71 64,25.71 63.2,26.51 63.2,28.16 64.08,29.05 v64.34,29.05
  Bottom 0.254: v64.34,29.05 64.08,28.8 R70.2
DY9_AMP_OUTP  (via drill 0.35)
  Top 0.203: IC10.13 68.06,25.15 67.17,24.27 66.78,24.27 C77.2 66.4,24.11 65.23,25.28 63.79,25.28 62.81,26.26 62.81,28.29 v64.34,29.82
  Bottom 0.254: v64.34,29.82 64.08,30.07 R74.2
DY9A  (via drill 0.35)
  Top 0.305: v42.41,26.12 41.52,26.12 D3.1 | D4.2 v37.71,38.05
  Bottom 0.305: R18.1 v42.41,26.12 C22.2 41.39,30.05 R4.2 R5.1 C23.1 v37.71,38.05
  pour Route15: 42.92,28.73 40.76,31.83 40.63,34.63 39.74,35.52 39.66,35.85 39.16,36.91 38.73,37.42 38.47,38.18 37.58,38.94 36.57,39.33 36.19,39.45 34.53,39.45 33.9,38.69 33.52,36.78 33.77,35.9 34.41,35.01 35.3,34.5 36.19,34.24 38.34,34.63 39.36,33.48 39.49,31.58 41.85,28.38 41.85,26.93 42.38,25.02 42.79,24.72 43.17,24.85 43.04,28.15
DY9B  (via drill 0.35)
  Top 0.305: v44.4,24.99 R40.1
  Bottom 0.305: R18.2 v44.4,24.99 C38.2
  pour Route15 (no thermals): 43.56,25.55 44.35,25.96 45.7,24.33 44.82,23.48 44.31,23.7 43.59,24.81
DY9C
  Top 0.305: C53.1 R46.1 43.77,28.55 R40.2
DY10
  Bottom 0.305: R45.2 DY10.P$1
  pour Route15 (no thermals): 47.58,19.78 48.97,20.16 49.48,20.16 49.73,19.78 49.72,18.65 49.47,18.34 49.11,18.17 47.01,18.12 46.17,18.27 45.25,20.25 45.29,20.93 46.05,21.31
DY10A  (via drill 0.35)
  Top 0.305: D2.1 v41.9,21.8 44.65,22.32 46.09,23.58 46.73,23.83 D1.A v48.84,25.12 | v39.49,29.04 D3.2
  Route15 0.508: v39.49,29.04 41.01,25.36 v41.9,21.8
  Bottom 0.305: C21.2 v41.9,21.8 41.98,21.77 R17.1 | C22.1 v39.49,29.04 R4.1 | R32.2 v48.84,25.12
  pour Route15: 36.46,31.91 37.33,26.75 37.73,26.19 40.63,25.36 40.88,23.7 40.07,21.9 40.05,20.83 40.25,20.5 41.04,20.38 42.36,21.24 42.34,22.42 41.52,24.47 41.01,26.62 41.01,28.02 39.99,29.29 37.84,31.83 37.58,33.23 37.2,33.48 36.69,33.48 36.44,33.23 36.44,32.85
  pour Route2 (no thermals): 49.1,25.37 48.59,25.37 47.7,24.1 47.96,22.32 48.97,22.32 49.23,22.83 49.23,24.23
DY10B  (via drill 0.35)
  Route15 0.305: v46.85,22.18 45.71,22.31 v43.98,20.82
  Bottom 0.305: R39.1 C37.2 v43.98,20.82 R17.2 | C38.1 v46.85,22.18 R38.2
  pour Route15 (no thermals): 42.28,20.02 42.28,19.39 42.53,19.13 43.8,19 44.95,18.24 45.58,18.24 45.58,18.5 44.57,20.02 44.57,21.29 43.8,21.29
  pour Route15: 46.85,22.43 48,22.18 49.01,22.18 49.01,21.16 48.76,20.78 48.25,20.78 46.47,22.05
DY10B_MON_A
  Bottom 0.305: R38.1 R37.2
DY10B_MON_B  (via drill 0.35)
  Top 0.203: v56.59,18.89 56.13,18.89 54.99,19.91 v54.48,20.8 | v88.44,21.1 89,21.66 91.03,21.66 91.31,21.94 93.4,21.94 94.39,22.93 94.64,22.93 v94.77,23.06
  Route15 0.203: v56.59,18.89 57.1,19.4 63.2,19.4 64.34,20.54 69.93,20.54 70.31,20.93 88.27,20.93 v88.44,21.1
  Bottom 0.203: v94.77,23.06 95.4,23.7 96.06,23.7 96.67,24.3 100.24,24.3 100.54,24.61 C51.1 101.05,25.75 R36.2
  Bottom 0.254: R37.1 v54.48,20.8
DY10C
  Bottom 0.305: C52.2 R45.1 46.81,18.51 R39.2
FPGA_C_!CS  (via drill 0.35)
  Top 0.152: IC9.16 89.66,27.42 90.19,26.89 93.24,26.89 97.01,30.66 v98.38,30.66 98.5,30.53 IC8.25
  Bottom 0.203: v98.38,30.66 98.32,30.66 R95.1
FPGA_CRESET_B  (via drill 0.35)
  Top 0.203: IC9.8 85.86,24.04 86.31,23.59 89.36,23.59 90.5,24.74 92.81,24.74 v93.14,25.07 | v101.8,32.1 101.7,31.99 IC8.21
  Bottom 0.152: v101.8,32.1 101.55,31.85 101.04,31.85 97.36,28.16 95.71,28.16 93.14,25.6 v93.14,25.07
FPGA_DRDY
  Top 0.152: IC9.13 89.13,25.92 89.3,25.75 93.7,25.75 96.5,28.55 99.5,28.55 IC8.29
FPGA_RESTART  (via drill 0.35)
  Top 0.203: IC9.12 87.86,25.09 87.99,24.97 89.11,24.97 89.41,25.27 v92.46,25.27 | v101.09,32.36 101.2,32.25 IC8.22
  Bottom 0.152: v101.09,32.36 101.09,32.33 97.28,28.52 95.43,28.52 92.46,25.55 v92.46,25.27
GND  (via drill 0.35, 0.5)
  Top 0.254: IC10.41 78.05,27.66 78.06,27.65 | IC8.49 105.2,25.53 IC8.47 105.2,23.68 105.21,23.7 | IC8.49 103.7,28.53 IC8.8 106.39,28.55 v107.9,28.55 | IC8.49 100.7,25.53 IC8.35 98.59,25.53 v98.5,25.62 | 105.21,23.21 v104.83,22.83 | IC8.49 102.86,27.78 100.7,29.95 IC8.23 100.7,31.94 100.38,32.25 100.38,32.83 100,33.21 C99.2
  Top 0.305: 78.06,27.65 78.38,27.65 | IC11.2 v104.98,20.93 | v95.38,17.9 IC13.2 | C123.2 92.84,17.28 v92.84,17.39 | R104.1 97.02,34.05 C121.1
  Top 0.406: 105.21,23.7 105.21,23.21 | C99.2 99.64,33.23 | v39.49,24.09 D2.2 | v34.28,22.18 34.28,24.97 C20.2 | v83.31,17.47 83.45,17.61 IC4.3 85.21,17.58 86.06,16.73 v86.31,16.73 | C131.1 104.72,33.87 v104.73,33.88 | J4.1 108.64,13.03 v108.66,13.05 | IC1.2 v36.82,19.26 | C18.2 28.85,17.39 C2.1 | R3.1 24.82,19.8 v25.31,19.56 | R2.1 51.64,27.61 v51.51,28.67 | C118.2 105.06,15.73 v105.06,14.91
  Top 0.508: 78.38,27.65 78.56,27.84 78.78,27.83 C105.2 79.42,27.82 79.88,28.29 v79.88,28.34 | v79.86,29.2 79.88,29.18 | v98.5,25.62 98.38,25.62 98.13,25.87 C88.2 | C85.2 105.44,23.01 105.06,23.01 104.93,22.88 104.83,22.88 v104.83,22.83 | 99.64,33.23 v99.64,33.88 99.48,34.05 C121.1 | C133.2 93.7,12.6 v93.6,12.7 | C124.2 98.09,13.85 v98.05,13.81 v98.04,13.81 C122.2 | v104.39,13.74 103.84,13.19 C127.2 | C109.2 91.29,32.25 v90.8,32.74 | C113.2 v109.04,17.88 | C93.2 109.01,29.15 108.41,28.55 v107.9,28.55 108.28,28.55 108.86,27.97 C94.2 | C19.2 24.88,27.13 v25.19,26.8 | J3.3 52.45,30.82 51.51,28.74 v51.51,28.67 | R60.2 55.45,29.13 55.45,31.77 | v101.88,20.82 101.81,20.76 C112.2
  Top 0.61: v55.45,33.24 55.45,31.77 J3.2 | C115.2 97.32,19.75 97.97,20.4 C114.2 99.26,20.4 | v34.84,17.41 v33.95,17.41 33.09,16.98 C1.1 C2.1 | J3.3 52.45,33.17 v52.53,33.24 | C64.1 86.54,16.5 v86.31,16.73 | C116.2 99.26,20.4 | 99.26,20.4 99.26,21.54 v99.21,21.59 | C58.2 72.88,15.88 v72.47,15.46 | v103.4,22.83 103.5,22.74 104.73,22.74 v104.83,22.83
  Top 0.762: 79.88,29.18 v79.88,28.34 79.88,28.39 v80.7,29.2 v79.86,29.2
  Route2 0.61: v71.2,33.75 70.56,33.8 65.48,33.8 61.2,33.02 59.27,32.72 v55.45,33.24 | v72.47,15.46 71.99,13.57 v70.05,12.8
  Route15 0.61: v98.05,13.81 97.27,14.58 95.52,14.58 95.11,14.18 91.16,14.17 90.88,14.45 v90.37,14.45
  Bottom 0.254: v102.95,29.18 98.86,29.18 97.11,27.43
  Bottom 0.305: C36.2 v51.51,28.67
  Bottom 0.406: IC12.2 95.84,30.68 | 95.84,30.68 95.84,30.45 C132.1 | 95.84,30.68 v95.89,30.63 96.45,30.07 R95.2 | v104.73,33.88 104.59,33.74 C34.2 102.49,33.74 R110.2 | C129.1 102.39,29.77 102.95,29.21 v102.95,29.18 | C21.1 v39.49,24.09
